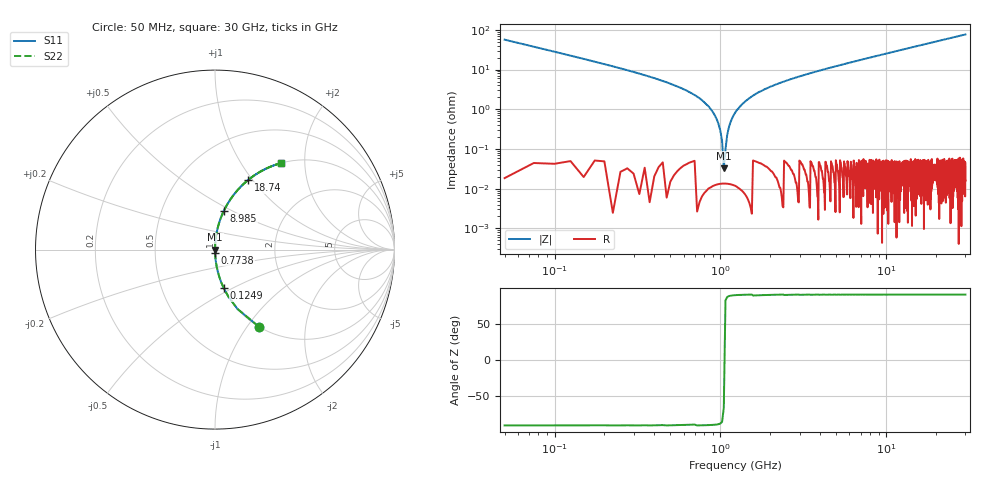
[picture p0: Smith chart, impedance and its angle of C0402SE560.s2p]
!	AVX Thin Film Operation 	Date: April 2014
!	Description: Accu-P® Series, Thin Film  SMD RF Capacitor
!	Part Number: 04023K560FBSTR
# MHZ S MA R 50
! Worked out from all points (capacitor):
!   1201 points, 50 MHz to 30 GHz, reference 50 ohm
!   read as one part in series: C = 56 pF near 199.8 MHz
!   lowest |Z| = 32.8 mohm at 1.048 GHz (marker M1)
!   series resonance near 1.054 GHz, so ESL is about 410 pH
!   S11 on the Smith chart (normalised r, x): 50 MHz: 1.00, -1.13; 124.9 MHz: 1.00, -0.45; 773.8 MHz: 1.00, -0.03; 8.985 GHz: 1.00, +0.45; 18.74 GHz: 1.00, +0.96; 30 GHz: 1.00, +1.53
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50  0.493 -60.4  0.87 29.6  0.87 29.6  0.493 -60.4
124.875  0.219 -77.3  0.975 12.6  0.975 12.6  0.219 -77.3
299.583  0.087 -84.8  0.996 5.0  0.996 5.0  0.087 -84.8
773.792  0.017 -88.1  1 1.0  1 1.0  0.017 -88.1
848.667  0.012 -88.0  1 0.7  1 0.7  0.012 -88.0
948.5  0.005713 -87.0  1 0.3  1 0.3  0.005713 -87.0
1048.333  0.0004047 -48.1  1 0.0  1 0.0  0.0004047 -48.1
1148.167  0.004615 86.4  1 -0.3  1 -0.3  0.004615 86.4
1198.083  0.00692 87.4  1 -0.4  1 -0.4  0.00692 87.4
1272.958  0.01 87.9  1 -0.6  1 -0.6  0.01 87.9
1447.667  0.017 88.1  1 -1.0  1 -1.0  0.017 88.1
1697.25  0.027 87.9  0.999 -1.5  0.999 -1.5  0.027 87.9
1996.75  0.037 87.5  0.999 -2.1  0.999 -2.1  0.037 87.5
3094.917  0.07 85.8  0.997 -4.0  0.997 -4.0  0.07 85.8
5041.667  0.122 82.8  0.992 -7.0  0.992 -7.0  0.122 82.8
8985.083  0.221 77.2  0.975 -12.8  0.975 -12.8  0.221 77.2
10058.29  0.246 75.7  0.969 -14.3  0.969 -14.3  0.246 75.7
15025  0.357 69.0  0.934 -20.9  0.934 -20.9  0.357 69.0
18743.79  0.431 64.4  0.902 -25.5  0.902 -25.5  0.431 64.4
20016.67  0.455 62.9  0.89 -27.0  0.89 -27.0  0.455 62.9
25033.29  0.538 57.4  0.842 -32.6  0.842 -32.6  0.538 57.4
30000  0.608 52.5  0.794 -37.5  0.794 -37.5  0.608 52.5
